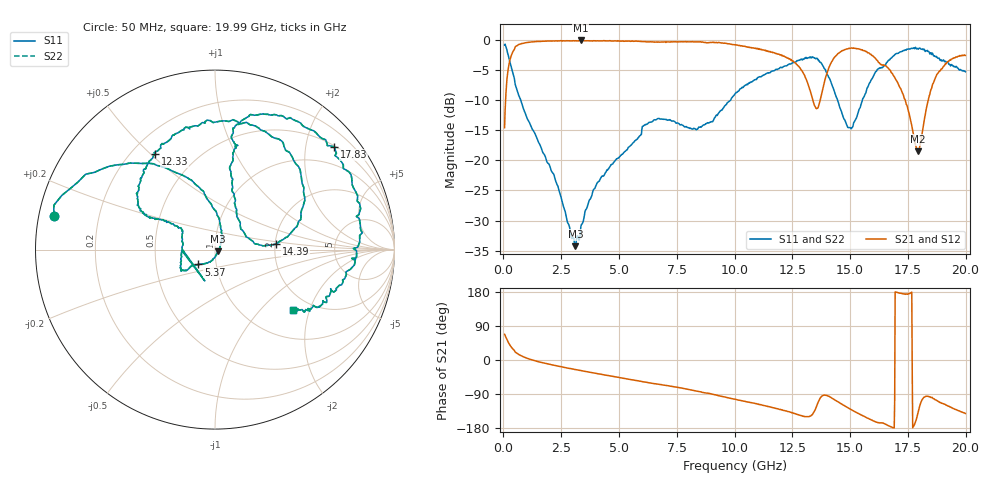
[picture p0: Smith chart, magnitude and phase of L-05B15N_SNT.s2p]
! Data Taken on a HP 8720C VNA using a shunt-through fixture with TRL* de-embedding
#	mhz	s	ma	r	50
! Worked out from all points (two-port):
!   998 points, 50 MHz to 19.99 GHz, reference 50 ohm
!   highest |S21| = 0.00 dB at 3.35 GHz (marker M1); lowest = -18.5 dB at 17.95 GHz (marker M2)
!   |S21| within 3 dB of the highest: 300.3 MHz to 12.34 GHz (12.04 GHz wide, 190 % of centre); 14.29 GHz to 16.1 GHz (1.813 GHz wide, 11.9 % of centre)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
!   lowest |S11| = -34.3 dB at 3.11 GHz (marker M3), VSWR 1.04, Z = 51.8 - j0.877 ohm
!   |S11| at or under -10 dB: 752.4 MHz to 9.819 GHz (9.067 GHz wide, 172 % of centre); 14.46 GHz to 15.53 GHz (1.066 GHz wide, 7.11 % of centre)
!   |S22| runs from -34.3 to -0.6 dB; largest |S21 - S12| = 0
!   S11 on the Smith chart (normalised r, x): 50 MHz: 0.04, +0.10; 5.37 GHz: 0.82, -0.14; 12.33 GHz: 0.29, +0.52; 14.39 GHz: 2.03, +0.15; 17.83 GHz: 0.53, +2.60; 19.99 GHz: 1.62, -1.55
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50  0.9181 168.3  0.1877 67.7  0.1877 67.7  0.9181 168.3
270  0.6753 134.4  0.6779 40.1  0.6779 40.1  0.6753 134.4
730  0.3254 100.8  0.933 12.3  0.933 12.3  0.3254 100.8
3110  0.01933 -26.0  0.9948 -25.2  0.9948 -25.2  0.01933 -26.0
3350  0.0281 -70.0  0.9995 -27.7  0.9995 -27.7  0.0281 -70.0
3390  0.02947 -71.9  0.9922 -28.4  0.9922 -28.4  0.02947 -71.9
5370  0.1242 -138.3  0.9875 -50.1  0.9875 -50.1  0.1242 -138.3
6710  0.2237 -147.8  0.97 -63.9  0.97 -63.9  0.2237 -147.8
8350  0.1804 172.0  0.9744 -81.7  0.9744 -81.7  0.1804 172.0
10030  0.3594 151.5  0.9186 -103.7  0.9186 -103.7  0.3594 151.5
12330  0.6301 122.1  0.7116 -136.4  0.7116 -136.4  0.6301 122.1
13350  0.7305 76.2  0.3395 -145.0  0.3395 -145.0  0.7305 76.2
13830  0.6095 37.2  0.403 -93.4  0.403 -93.4  0.6095 37.2
14390  0.342 5.4  0.746 -107.3  0.746 -107.3  0.342 5.4
15050  0.1837 38.2  0.8667 -131.2  0.8667 -131.2  0.1837 38.2
15750  0.4054 75.8  0.7906 -153.5  0.7906 -153.5  0.4054 75.8
16670  0.6853 81.5  0.5819 -173.8  0.5819 -173.8  0.6853 81.5
17310  0.8252 65.5  0.3494 174.6  0.3494 174.6  0.8252 65.5
17830  0.8769 40.7  0.1358 -162.8  0.1358 -162.8  0.8769 40.7
17950  0.8459 32.3  0.1194 -137.0  0.1194 -137.0  0.8459 32.3
18750  0.7327 -15.5  0.5188 -106.8  0.5188 -106.8  0.7327 -15.5
19990  0.5482 -37.6  0.7502 -141.0  0.7502 -141.0  0.5482 -37.6
